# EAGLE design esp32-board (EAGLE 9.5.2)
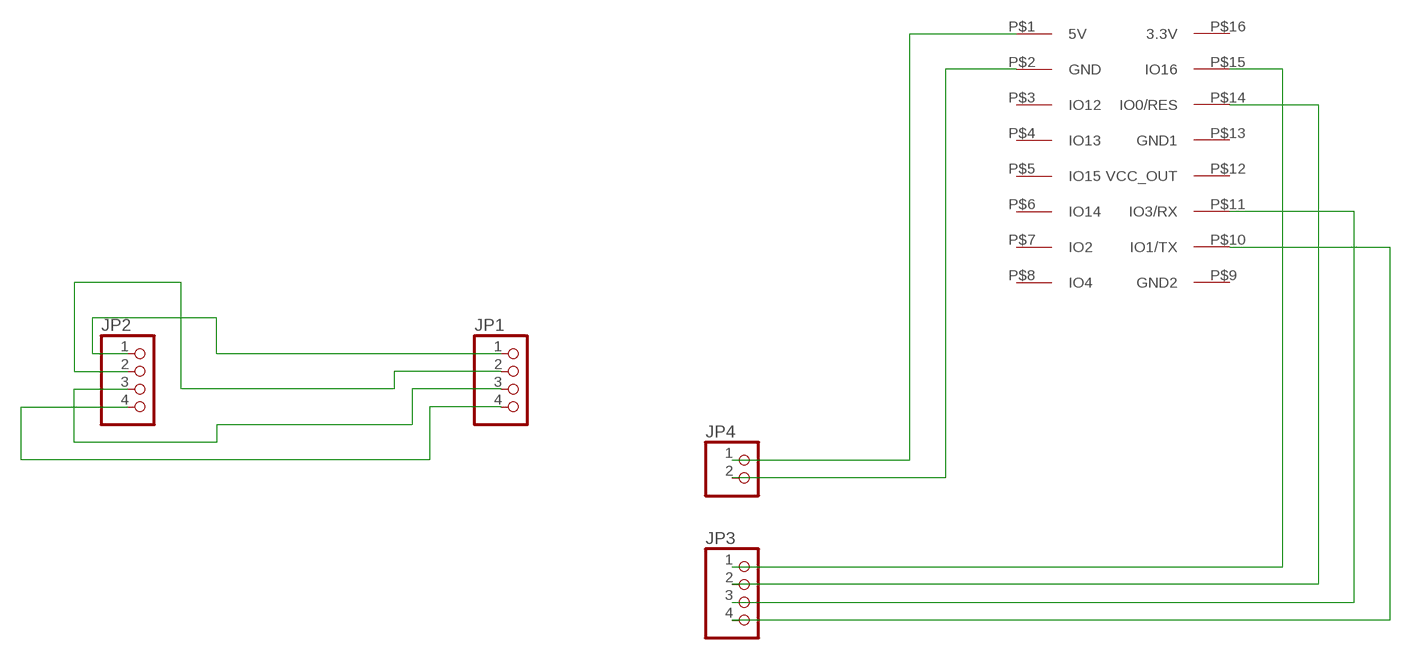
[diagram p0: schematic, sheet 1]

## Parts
JP1  PINHD-1X4  [1X04]
JP2  PINHD-1X4  [1X04]
JP3  PINHD-1X4  [1X04]
JP4  PINHD-1X2  [1X02]
U$3  ESP32-CAM  [ESP32-CAM_SMD]

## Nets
N$1: JP4.1 U$3.P$1(5V)
N$2: JP4.2 U$3.P$2(GND)
N$3: JP3.1 U$3.P$15(IO16)
N$4: JP3.2 U$3.P$14(IO0/RES)
N$5: JP3.3 U$3.P$11(IO3/RX)
N$6: JP3.4 U$3.P$10(IO1/TX)
N$7: JP1.1 JP2.1
N$8: JP1.2 JP2.2
N$9: JP1.3 JP2.3
N$14: JP1.4 JP2.4
Unconnected: U$3.P$3(IO12) U$3.P$4(IO13) U$3.P$5(IO15) U$3.P$6(IO14) U$3.P$7(IO2) U$3.P$8(IO4) U$3.P$9(GND2) U$3.P$12(VCC_OUT) U$3.P$13(GND1) U$3.P$16(3.3V)

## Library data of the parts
JP1-JP3 = pinhead:PINHD-1X4: PIN HEADER
JP4 = pinhead:PINHD-1X2: PIN HEADER
U$3 = ESP32-CAM:ESP32-CAM

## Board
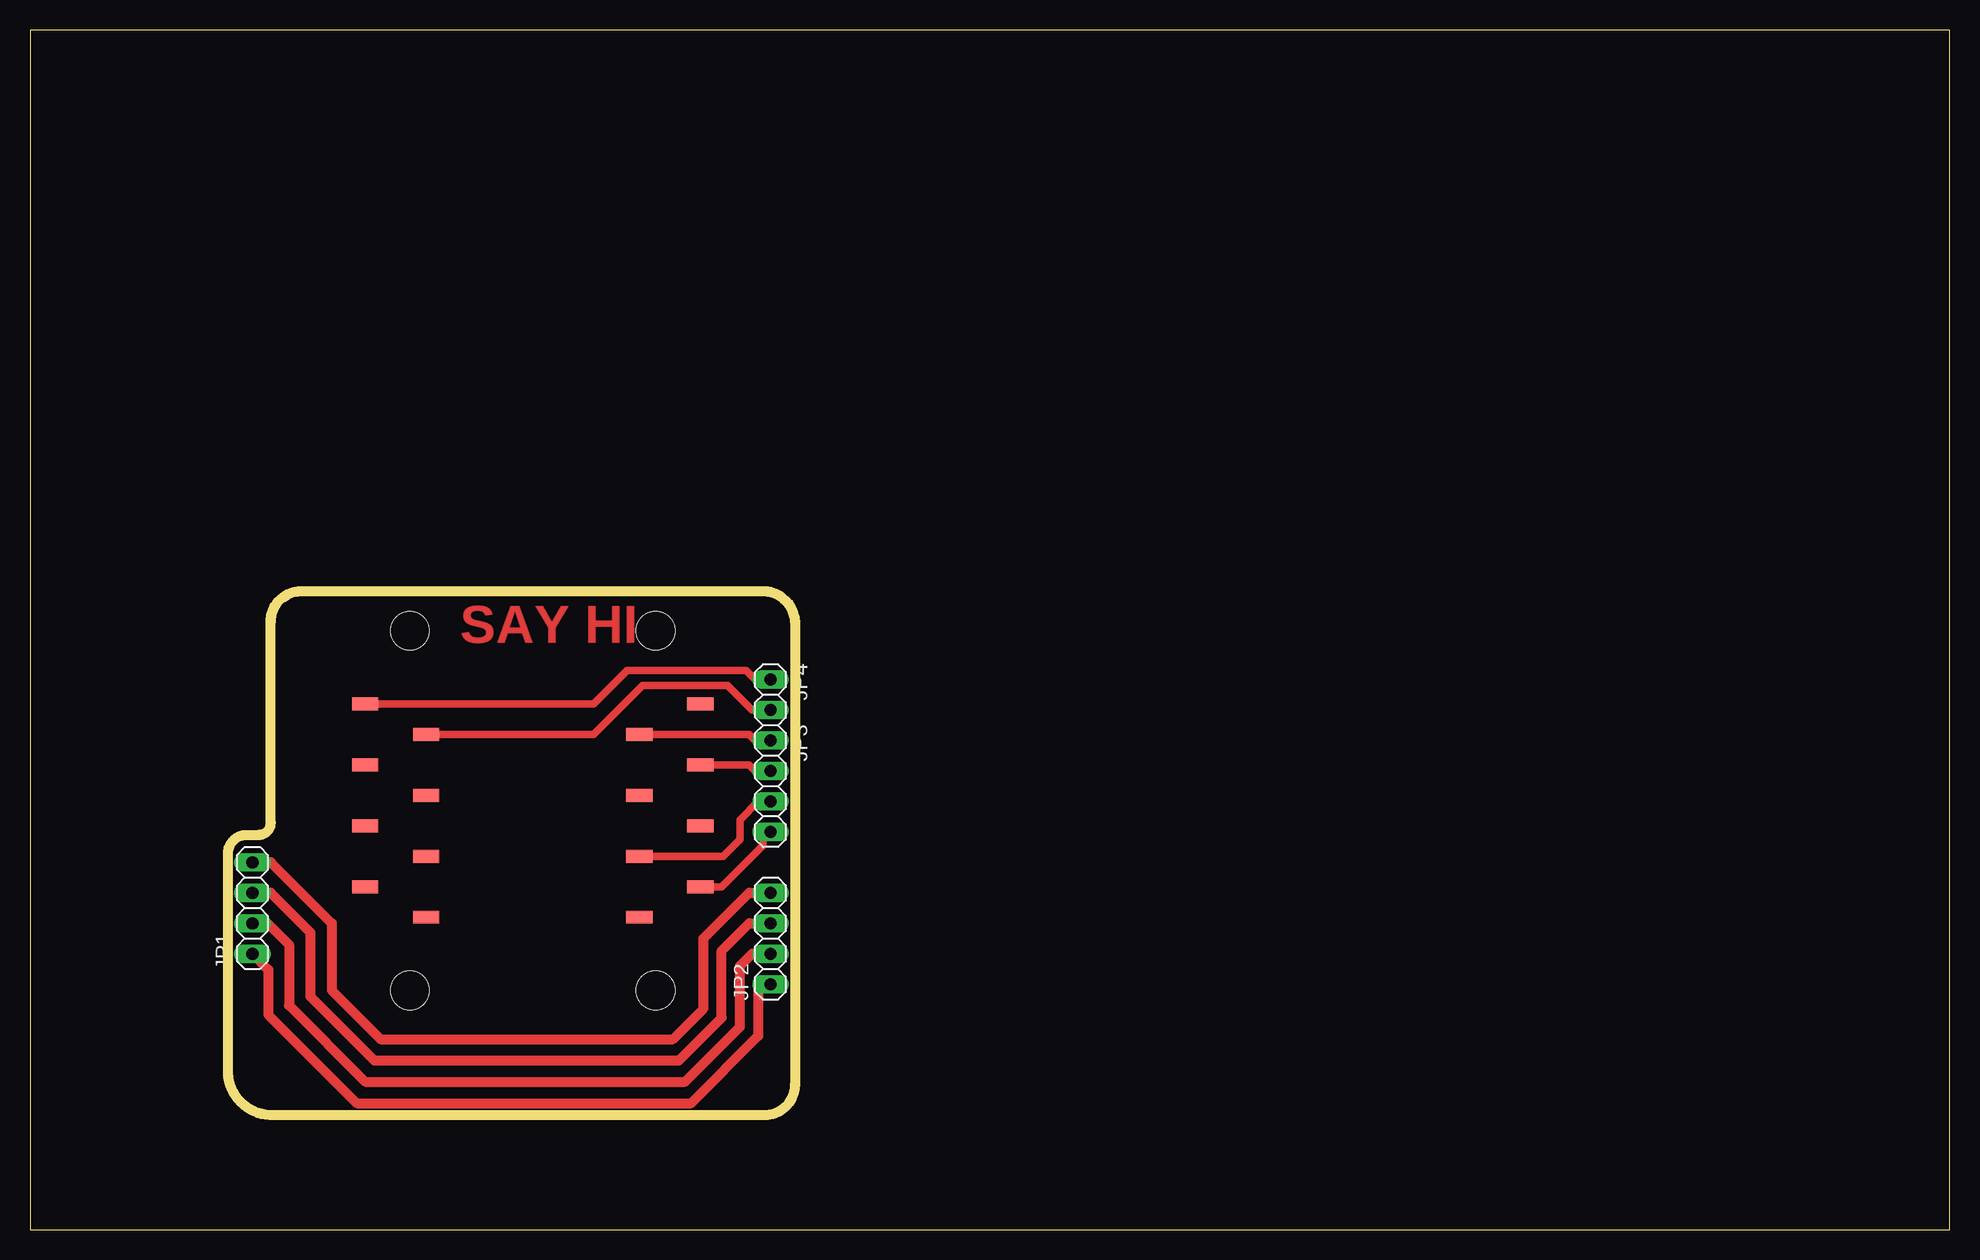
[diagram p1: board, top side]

Size 160 x 100 mm. Coordinates in mm from the lower left corner, seen from the top.
Outline: 0,0 160,0 160,100 0,100 0,0
Copper layers (1*16): Top 0.035mm / dielectric 1.5mm / Bottom 0.035mm
Design rules "default *": minimum track width 6mil, minimum drill 0.35mm, track to track 16mil, track to pad 16mil, pad to pad 16mil, via to via 16mil, smd to smd 16mil, copper to edge 40mil, drill to drill 6mil, minimum pad ring 10mil, minimum via ring 8mil, stop-mask expansion 4mil, vias tented up to drill 0mil, thermal gap 10mil
Holes 3.2 mm at 31.67,19.94 52.15,19.94 52.15,49.91 31.67,49.91
Milling: 12 lines

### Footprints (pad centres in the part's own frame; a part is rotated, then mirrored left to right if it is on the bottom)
1X04 = drill 1.016 long: 1 -3.81,0; 2 -1.27,0; 3 1.27,0; 4 3.81,0
1X02 = drill 1.016 long: 1 -1.27,0; 2 1.27,0
ESP32-CAM_SMD = smd 2.184 x 1.067: P$1 -13.97,8.89; P$2 -8.89,6.35; P$3 -13.97,3.81; P$4 -8.89,1.27; P$5 -13.97,-1.27; P$6 -8.89,-3.81; P$7 -13.97,-6.35; P$8 -8.89,-8.89; P$9 8.89,-8.89; P$10 13.97,-6.35; P$11 8.89,-3.81; P$12 13.97,-1.27; P$13 8.89,1.27; P$14 13.97,3.81; P$15 8.89,6.35; P$16 13.97,8.89

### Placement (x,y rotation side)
JP1  18.54,26.8 90 top
JP2  61.72,24.26 90 top
JP3  61.72,36.96 270 top
JP4  61.72,44.58 270 top
U$3  41.91,34.92 0 top

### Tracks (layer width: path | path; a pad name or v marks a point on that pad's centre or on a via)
N$1
  Top 0.61: U$3.P$1 46.99,43.81 49.78,46.61 59.69,46.61 60.45,45.85 JP4.1
N$2
  Top 0.61: U$3.P$2 46.99,41.27 51.05,45.34 58.17,45.34 60.2,43.31 JP4.2
N$3
  Top 0.61: JP3.1 60.45,40.77 59.94,41.27 U$3.P$15
N$4
  Top 0.61: JP3.2 60.45,38.23 59.94,38.73 U$3.P$14
N$5
  Top 0.61: U$3.P$11 57.78,31.11 59.18,32.51 59.18,34.16 60.71,35.69 JP3.3
N$6
  Top 0.61: U$3.P$10 57.66,28.57 61.09,32 61.09,32.64 61.21,32.64 JP3.4
N$7
  Top 0.813: JP1.1 19.86,21.67 19.86,17.91 27.23,10.54 55.12,10.54 60.71,16.13 60.71,20.19 60.96,20.45 JP2.1
N$8
  Top 0.813: JP1.2 19.81,25.53 21.59,23.75 21.59,18.67 27.94,12.32 54.61,12.32 59.18,16.89 59.18,21.97 60.2,22.99 JP2.2
N$9
  Top 0.813: JP1.3 20.07,28.07 23.37,24.76 23.37,19.43 28.7,14.1 54.1,14.1 57.66,17.65 57.66,23.24 59.94,25.53 JP2.3
N$14
  Top 0.813: JP1.4 20.07,30.61 25.15,25.53 25.15,19.94 29.21,15.87 53.59,15.87 56.13,18.41 56.13,24.26 59.94,28.07 JP2.4

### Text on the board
Top: SAY HI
